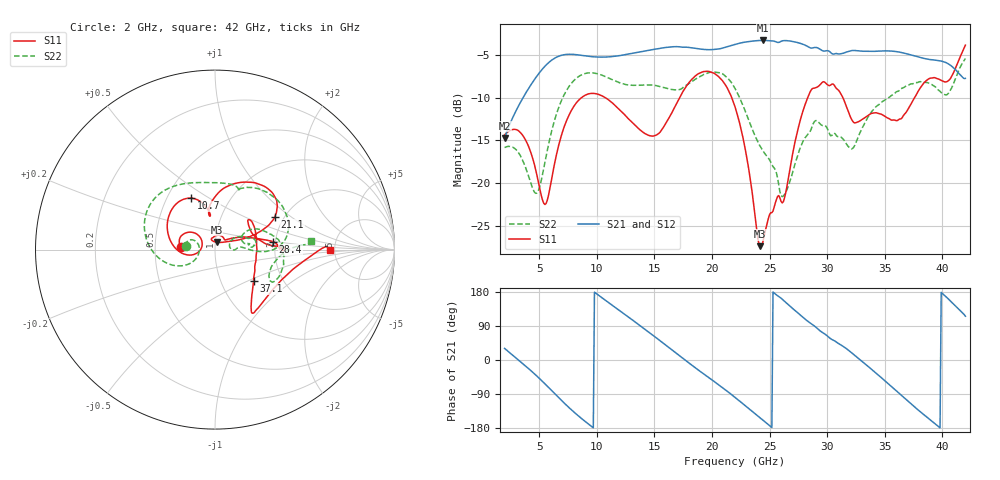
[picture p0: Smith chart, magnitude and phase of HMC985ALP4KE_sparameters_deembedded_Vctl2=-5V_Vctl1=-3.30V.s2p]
!s2p File: Measurements: S11, S21, S12, S22
# GHz S dB R 50.0
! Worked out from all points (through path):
!   401 points, 2 GHz to 42 GHz, reference 50 ohm
!   highest |S21| = -3.33 dB at 24.4 GHz (marker M1); lowest = -14.7 dB at 2 GHz (marker M2)
!   lowest |S11| = -27.4 dB at 24.2 GHz (marker M3), VSWR 1.09, Z = 50.7 + j4.25 ohm
!   |S11| at or under -10 dB: start of sweep to 8.688 GHz; 10.72 GHz to 17.2 GHz (6.488 GHz wide, 46.5 % of centre); 21.71 GHz to 28.32 GHz (6.604 GHz wide, 26.4 % of centre)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
!   |S22| runs from -21.6 to -5.4 dB; largest |S21 - S12| = 0.00063
!   S11 on the Smith chart (normalised r, x): 2 GHz: 0.68, +0.02; 10.7 GHz: 0.66, +0.42; 21.1 GHz: 1.79, +0.77; 28.4 GHz: 1.95, +0.19; 37.1 GHz: 1.43, -0.54; 42 GHz: 4.56, +0.01
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2  -14.37 176.2  -14.72 30.6  -14.73 30.6  -15.85 173.0
4.7  -18.47 139.5  -7.69 -39.6  -7.69 -39.6  -21.21 177.6
5.5  -22.52 166.5  -6.34 -62.8  -6.35 -62.8  -17.58 -152.1
6.9  -14.57 -174.1  -5.08 -105.5  -5.08 -105.5  -10.46 -168.1
8.7  -9.99 144.7  -5.07 -155.0  -5.08 -155.0  -7.33 154.5
10.7  -9.99 115.1  -5.27 158.7  -5.27 158.7  -7.53 122.7
13.3  -13.20 99.2  -4.78 101.0  -4.79 101.0  -8.57 87.7
15.4  -14.19 99.9  -4.28 53.1  -4.28 53.1  -8.69 70.1
18  -8.27 72.9  -4.14 -7.8  -4.14 -7.8  -8.36 64.6
21.1  -8.40 28.7  -4.15 -77.0  -4.15 -77.0  -7.42 15.8
22  -11.08 22.1  -3.79 -98.6  -3.79 -98.5  -8.94 3.0
24.2  -27.39 78.6  -3.33 -153.0  -3.33 -153.0  -15.74 3.4
24.4  -27.01 96.4  -3.33 -158.0  -3.32 -158.0  -16.20 4.5
26.2  -22.18 43.5  -3.35 157.7  -3.35 157.7  -21.52 16.1
28.4  -9.71 7.7  -4.09 100.3  -4.10 100.3  -14.21 18.6
28.7  -8.97 2.8  -4.21 94.3  -4.22 94.3  -13.37 17.5
30.6  -8.53 1.4  -4.92 51.4  -4.92 51.4  -14.16 9.7
32.4  -12.98 26.0  -4.50 11.9  -4.50 12.0  -15.58 26.0
35.4  -12.49 12.8  -4.55 -65.4  -4.55 -65.3  -9.96 16.0
37.1  -11.17 -38.9  -4.96 -111.1  -4.96 -111.0  -8.52 2.0
39.7  -7.86 -53.7  -5.68 -176.5  -5.68 -176.5  -9.17 -29.3
42  -3.87 0.0  -7.76 115.6  -7.77 115.6  -5.43 5.4
